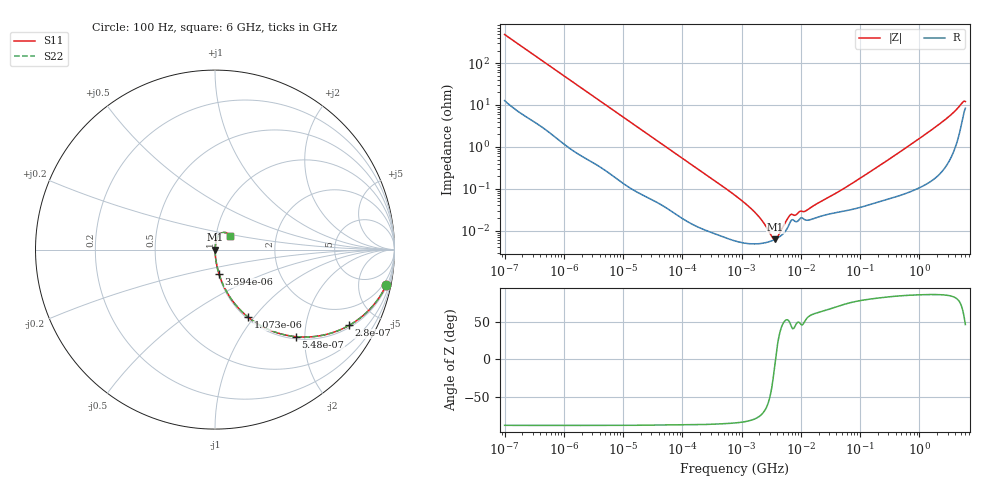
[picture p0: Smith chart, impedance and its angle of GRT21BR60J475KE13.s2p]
!Murata Part Number: GRT21BR60J475KE13
!These Parameters are Measured in Series Mode Connection
!Data Generated on Jun 19, 2026
!  o--ll--o
!Port1  Port2
!  o------o
!Operation Temp=25[degC], DC Bias Voltage=0[V]
!Freq. Start=100[Hz] Stop=6[GHz] 401[Steps]
# Hz S RI R 50
!Freq.(Hz) S11(Real) S11(Imag) S21(Real) S21(Imag) S12(Real) S12(Imag) S22(Real) S22(Imag)
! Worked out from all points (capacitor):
!   401 points, 100 Hz to 6 GHz, reference 50 ohm
!   read as one part in series: C = 3.28 uF near 109 Hz
!   lowest |Z| = 6.26 mohm at 3.712 MHz (marker M1)
!   series resonance near 3.745 MHz, so ESL is about 550 pH
!   S11 on the Smith chart (normalised r, x): 100 Hz: 1.25, -9.66; 280 Hz: 1.09, -3.50; 548 Hz: 1.05, -1.81; 1.073 kHz: 1.02, -0.93; 3.594 kHz: 1.01, -0.28; 6 GHz: 1.17, +0.18
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100  0.9542 -0.1963  0.0458 0.1963  0.0458 0.1963  0.9542 -0.1963
164  0.8924 -0.2979  0.1076 0.2979  0.1076 0.2979  0.8924 -0.2979
280  0.7481 -0.4217  0.2519 0.4217  0.2519 0.4217  0.7481 -0.4217
548  0.4509 -0.485  0.5491 0.485  0.5491 0.485  0.4509 -0.485
1073  0.1843 -0.3763  0.8157 0.3763  0.8157 0.3763  0.1843 -0.3763
2008  0.0642 -0.2335  0.9358 0.2335  0.9358 0.2335  0.0642 -0.2335
3594  0.0231 -0.1378  0.9769 0.1378  0.9769 0.1378  0.0231 -0.1378
9626  0.00427 -0.0535  0.9957 0.0535  0.9957 0.0535  0.00427 -0.0535
40335  0.000618 -0.0131  0.9994 0.0131  0.9994 0.0131  0.000618 -0.0131
774597  5.73e-05 -0.000695  0.9999 0.000695  0.9999 0.000695  5.73e-05 -0.000695
1658239  4.83e-05 -0.000275  1 0.000275  1 0.000275  4.83e-05 -0.000275
2837864  5.38e-05 -8.54e-05  0.9999 8.54e-05  0.9999 8.54e-05  5.38e-05 -8.54e-05
3712478  6.25e-05 -2.6e-06  0.9999 2.6e-06  0.9999 2.6e-06  6.25e-05 -2.6e-06
4643984  7.62e-05 6.74e-05  0.9999 -6.74e-05  0.9999 -6.74e-05  7.62e-05 6.74e-05
6644369  0.000161 0.000176  0.9998 -0.000176  0.9998 -0.000176  0.000161 0.000176
1.189169e7  0.00018 0.000229  0.9998 -0.000229  0.9998 -0.000229  0.00018 0.000229
1.555665e7  0.000189 0.000324  0.9998 -0.000324  0.9998 -0.000324  0.000189 0.000324
5.699437e7  0.000299 0.00103  0.9997 -0.00103  0.9997 -0.00103  0.000299 0.00103
3.124326e8  0.000603 0.00509  0.9994 -0.00509  0.9994 -0.00509  0.000603 0.00509
3.505958e9  0.00939 0.059  0.9906 -0.059  0.9906 -0.059  0.00939 0.059
5.245841e9  0.0472 0.0955  0.9528 -0.0955  0.9528 -0.0955  0.0472 0.0955
6e9  0.0833 0.0743  0.9167 -0.0743  0.9167 -0.0743  0.0833 0.0743
